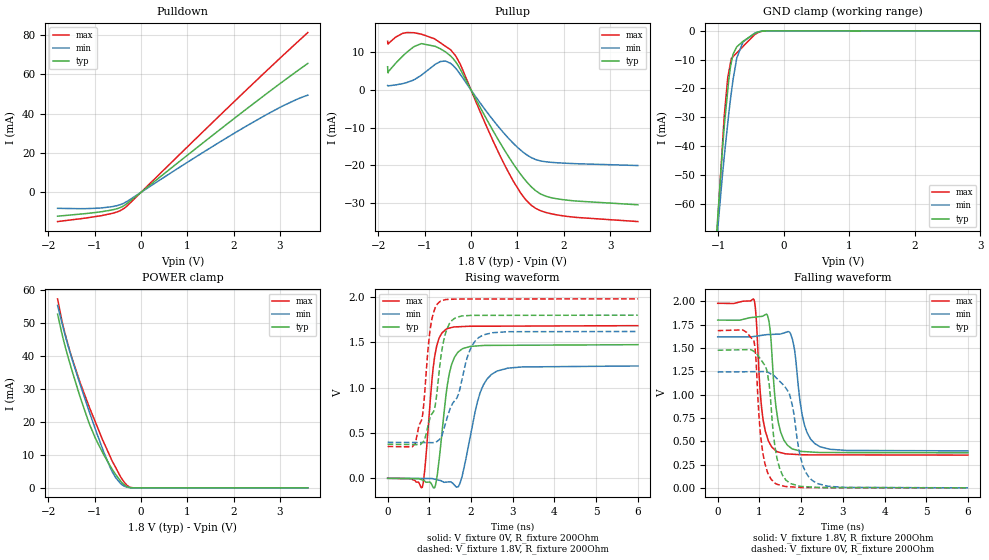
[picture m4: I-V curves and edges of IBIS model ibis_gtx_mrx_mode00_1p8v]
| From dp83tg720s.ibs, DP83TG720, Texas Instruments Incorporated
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| ibis_gtx_mrx_mode00_1p8v
[Model]   ibis_gtx_mrx_mode00_1p8v
Model_type   I/O
Polarity   Non-Inverting
Enable   Active-Low
Vinl = 0.54
Vinh = 1.26
Vmeas = 0.9
Vref = 0.9
Cref = 2pF
Rref = 100000
|   typ   min   max
C_comp   2.91pF   2.88pF   2.94pF
[Voltage Range]   1.8   1.62   1.98
[Temperature Range]   27   150   -40
[Pullup Reference]   1.8   1.62   1.98
[Pulldown Reference]   0   0   0
[Power Clamp Reference]   1.8   1.62   1.98
[GND Clamp Reference]   0   0   0
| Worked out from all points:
|   slope of the pulldown table from 0 to 0.27 V, typ, clamps not added: 52.7 ohm
|   slope of the pullup table from 0 to 0.27 V, typ, clamps not added: 43.2 ohm
|   GND clamp passes 1 mA (typ) near -0.45 V on its own axis
|   POWER clamp passes 1 mA (typ) near -0.37 V on its own axis
|   falling waveform, V_fixture 1.8V, R_fixture 200Ohm: 20-80 % time 187ps typ, 233ps min, 167ps max; typ from 1.8 V to 0.376 V
|   rising waveform, V_fixture 0V, R_fixture 200Ohm: 20-80 % time 235ps typ, 369ps min, 194ps max; typ from 0 V to 1.47 V
|   rising waveform, V_fixture 1.8V, R_fixture 200Ohm: 20-80 % time 330ps typ, 531ps min, 194ps max; typ from 0.376 V to 1.8 V
|   falling waveform, V_fixture 0V, R_fixture 200Ohm: 20-80 % time 224ps typ, 306ps min, 177ps max; typ from 1.48 V to 0 V
[Pulldown]
|   Voltage   I(typ)   I(min)   I(max)
-1.8V     -12.14mA   -8.138mA   -14.87mA
-1.217V   -10.87mA   -8.307mA   -13.16mA
-855mV    -9.881mA   -7.938mA   -11.87mA
-520.2mV  -8.35mA    -6.791mA   -10.01mA
-358.2mV  -6.641mA   -5.371mA   -8.07mA
1.165V    21.93mA    17.72mA    26.86mA
2.25V     41.92mA    33.37mA    51.53mA
3.065V    56.45mA    43.99mA    69.67mA
3.6V      65.57mA    49.42mA    81.25mA
[GND Clamp]
|   Voltage   I(typ)   I(min)   I(max)
-1.8V     -380.2mA   -330.5mA   -422.8mA
-1.017V   -67.69mA   -70.97mA   -69.38mA
-903.6mV  -31.87mA   -42.44mA   -28.15mA
-855mV    -20.52mA   -32.01mA   -16.18mA
-838.8mV  -16.74mA   -28.53mA   -14.19mA
-801mV    -11mA      -21.47mA   -9.556mA
-774mV    -8.056mA   -16.83mA   -8.932mA
-714.6mV  -5.478mA   -9.212mA   -7.557mA
-622.8mV  -3.648mA   -3.867mA   -5.433mA
-444.6mV  -916.7uA   -819.7uA   -1.31mA
-261mV    -11.9uA    -29.84uA   -11.43uA
3.6V      0A         0A         0A
[Pullup]
|   Voltage   I(typ)   I(min)   I(max)
-1.8V     6.185mA    1.233mA    12.95mA
-1.789V   4.544mA    1.116mA    12.24mA
-1.476V   9.02mA     1.707mA    15.04mA
-1.076V   12.31mA    3.899mA    14.84mA
-660.6mV  10.95mA    7.565mA    12.54mA
-444.6mV  9.078mA    7.111mA    10.73mA
-239.4mV  5.65mA     4.28mA     7.036mA
343.8mV   -7.913mA   -5.854mA   -9.914mA
797.4mV   -17.43mA   -12.65mA   -21.6mA
1.305V    -25.73mA   -17.95mA   -30.62mA
1.845V    -28.84mA   -19.28mA   -33.11mA
3.6V      -30.44mA   -20.03mA   -34.9mA
[POWER Clamp]
|   Voltage   I(typ)   I(min)   I(max)
-1.8V     52.72mA    55.38mA    57.36mA
-1.681V   45.36mA    48.69mA    49.19mA
-1.546V   38.34mA    41.79mA    42.08mA
-1.319V   27.84mA    31.66mA    32.21mA
-1.114V   19.41mA    23.05mA    24.46mA
-979.2mV  14.91mA    17.57mA    19.78mA
-811.8mV  10.26mA    11.13mA    14.04mA
-612mV    5.438mA    4.663mA    7.891mA
-444.6mV  2.133mA    1.367mA    3.461mA
-293.4mV  326.9uA    184.7uA    674.2uA
-109.8mV  6.036uA    6.315uA    2.646uA
3.6V      0A         0A         0A
[Ramp]
R_load = 200
|   typ   min   max
dV/dt_r   0.884663/2.33297e-10   0.743738/3.66249e-10   1.01063/1.93582e-10
dV/dt_f   0.854478/1.83763e-10   0.733764/2.30014e-10   0.977076/1.64042e-10
[Falling Waveform]
V_fixture = 1.8V
V_fixture_min = 1.62V
V_fixture_max = 1.98V
R_fixture = 200Ohm
C_fixture = 0F
|   Time   V(typ)   V(min)   V(max)
0s        1.8V       1.62V      1.98V
869.2ps   1.831V     1.624V     2.02V
922.8ps   1.833V     1.628V     1.825V
1.05ns    1.84V      1.636V     874.9mV
1.204ns   1.837V     1.645V     522mV
1.399ns   866.2mV    1.649V     395.6mV
1.751ns   430mV      1.648V     361.8mV
2.073ns   389.1mV    687.2mV    354.1mV
2.449ns   379.3mV    442mV      353.9mV
6ns       375.8mV    397mV      351.5mV
[Rising Waveform]
V_fixture = 0V
V_fixture_min = 0V
V_fixture_max = 0V
R_fixture = 200Ohm
C_fixture = 0F
|   Time   V(typ)   V(min)   V(max)
0s        1.917uV    11.86uV    845nV
829.6ps   -17.4mV    -1.986mV   -100.8mV
888.3ps   -30.71mV   -2.127mV   84.76mV
1.135ns   -95.95mV   -9.927mV   1.361V
1.399ns   916.1mV    -42.34mV   1.643V
1.535ns   1.258V     -46.18mV   1.664V
1.735ns   1.409V     -55.25mV   1.673V
2.208ns   1.463V     929.9mV    1.678V
2.621ns   1.467V     1.183V     1.679V
6ns       1.474V     1.24V      1.684V
[Rising Waveform]
V_fixture = 1.8V
V_fixture_min = 1.62V
V_fixture_max = 1.98V
R_fixture = 200Ohm
C_fixture = 0F
|   Time   V(typ)   V(min)   V(max)
0s        375.8mV    397mV      351.5mV
659.3ps   372.3mV    394.9mV    384.7mV
841.5ps   398.3mV    394.3mV    711.2mV
1.044ns   697.9mV    393.7mV    1.715V
1.142ns   807mV      393.4mV    1.883V
1.266ns   1.299V     441.8mV    1.955V
1.545ns   1.744V     814.7mV    1.976V
1.977ns   1.797V     1.419V     1.978V
2.282ns   1.798V     1.579V     1.979V
6ns       1.8V       1.62V      1.98V
[Falling Waveform]
|Gnd
V_fixture = 0V
V_fixture_min = 0V
V_fixture_max = 0V
R_fixture = 200Ohm
C_fixture = 0F
|   Time   V(typ)   V(min)   V(max)
0s        1.477V     1.243V     1.687V
861.1ps   1.466V     1.247V     1.588V
1.076ns   1.35V      1.248V     392.1mV
1.234ns   1.107V     1.233V     130.2mV
1.381ns   423mV      1.191V     48.33mV
1.632ns   84.76mV    1.072V     13.94mV
1.793ns   39.76mV    878.5mV    9.653mV
2.039ns   14.32mV    242.5mV    3.088mV
2.38ns    5.045mV    48.09mV    2.588mV
6ns       1.994uV    11.85uV    770.5nV
